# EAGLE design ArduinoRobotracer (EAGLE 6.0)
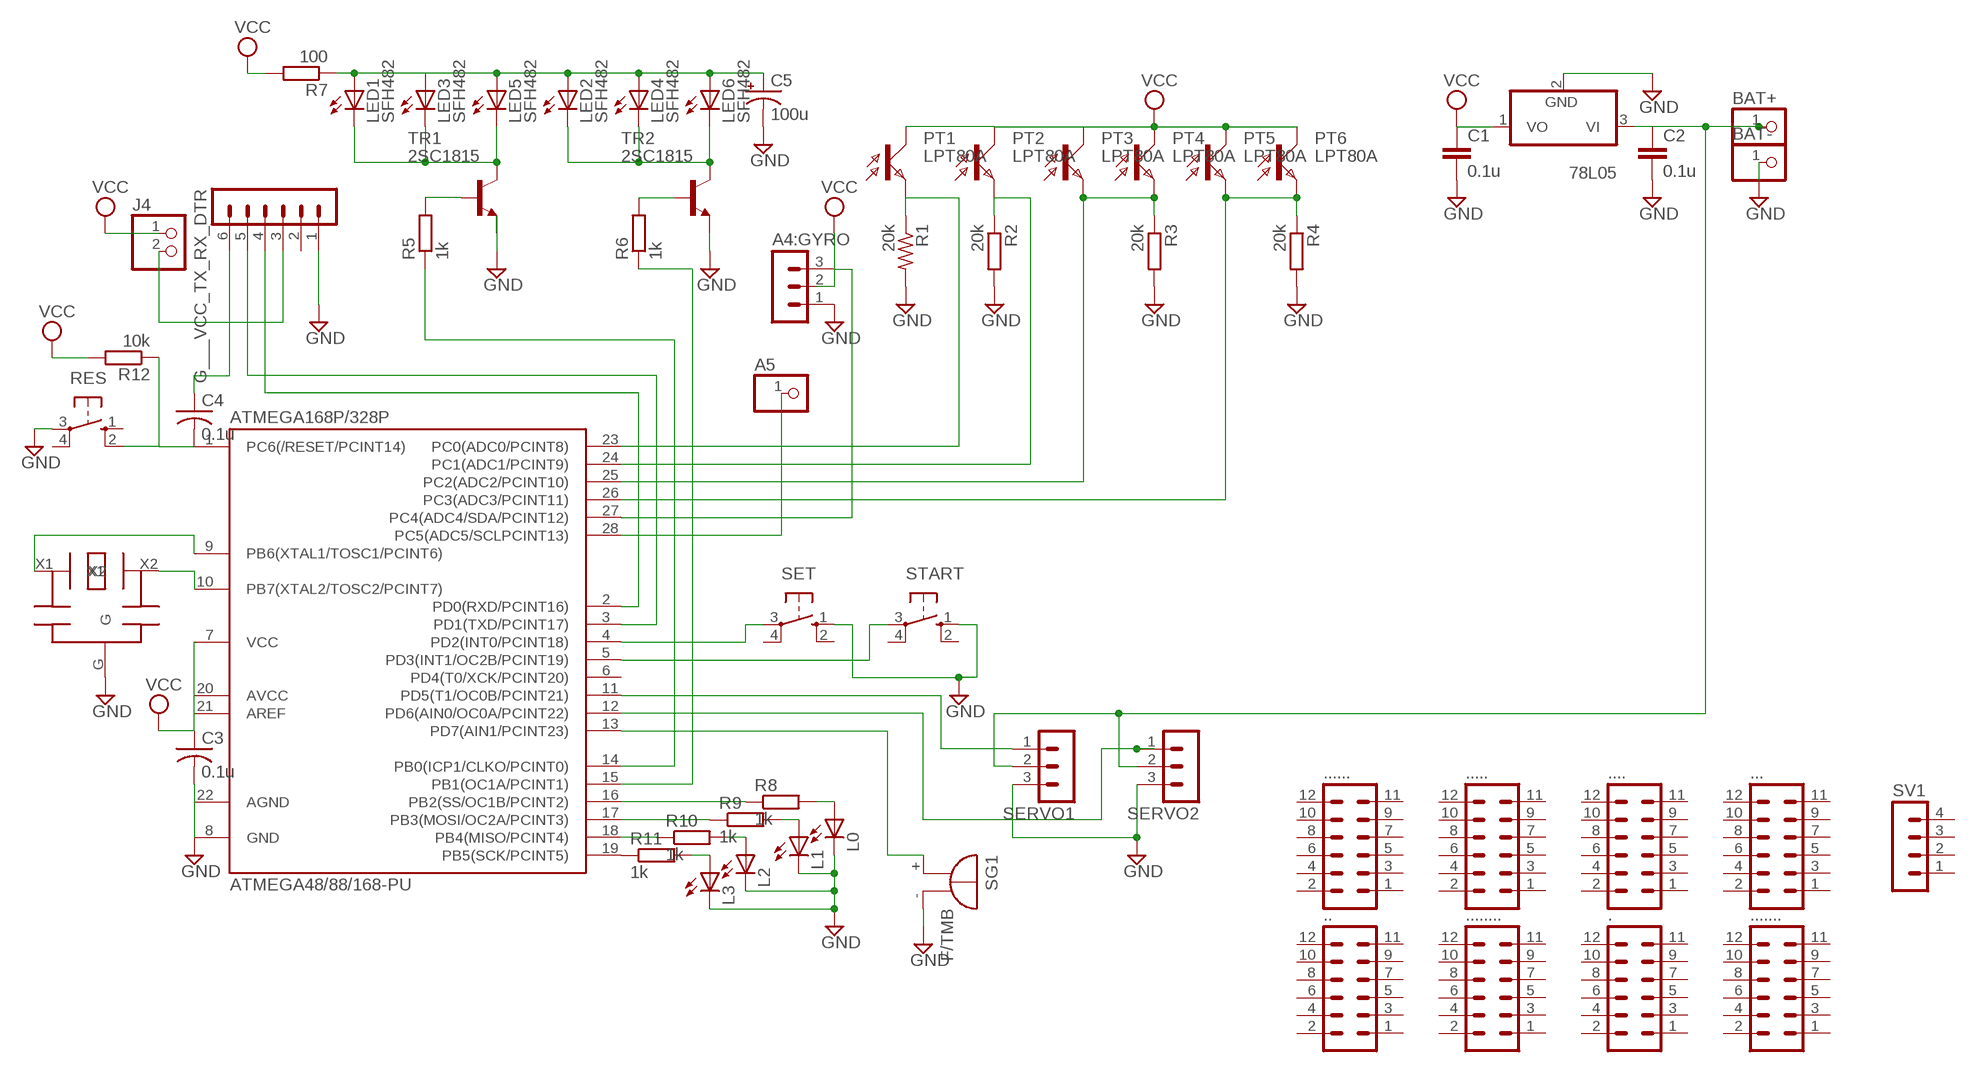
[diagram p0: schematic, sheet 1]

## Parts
78L05  78L05  [TO92-]
.  MA06-2  [MA06-2]
..  MA06-2  [MA06-2]
...  MA06-2  [MA06-2]
....  MA06-2  [MA06-2]
.....  MA06-2  [MA06-2]
......  MA06-2  [MA06-2]
.......  MA06-2  [MA06-2]
........  MA06-2  [MA06-2]
A4:GYRO  MA03-1  [MA03-1]
A5  PINHD-1X1  [1X01]
ATMEGA168P/328P  ATMEGA48/88/168-PU  [DIL28-3]
BAT+  PINHD-1X1  [1X01]
BAT-  PINHD-1X1  [1X01]
C1  0.1u  C2.5/2  [C2.5-2]
C2  0.1u  C2.5/2  [C2.5-2]
C3  0.1u  C-US025-025X050  [C025-025X050]
C4  0.1u  C-US025-025X050  [C025-025X050]
C5  100u  CPOL-USTT2D5  [TT2D5]
G___VCC_TX_RX_DTR  MA06-1  [MA06-1]
J4  PINHD-1X2  [1X02]
L0  LED3MM  [LED3MM]
L1  LED3MM  [LED3MM]
L2  LED3MM  [LED3MM]
L3  LED3MM  [LED3MM]
LED1  SFH482  [SFH482]
LED2  SFH482  [SFH482]
LED3  SFH482  [SFH482]
LED4  SFH482  [SFH482]
LED5  SFH482  [SFH482]
LED6  SFH482  [SFH482]
PT1  LPT80A  [LPT80A]
PT2  LPT80A  [LPT80A]
PT3  LPT80A  [LPT80A]
PT4  LPT80A  [LPT80A]
PT5  LPT80A  [LPT80A]
PT6  LPT80A  [LPT80A]
R1  20k  R-US_0204/2V  [0204V]
R2  20k  R-EU_0204/2V  [0204V]
R3  20k  R-EU_0204/2V  [0204V]
R4  20k  R-EU_0204/2V  [0204V]
R5  1k  R-EU_0204/2V  [0204V]
R6  1k  R-EU_0204/2V  [0204V]
R7  100  R-EU_0204/2V  [0204V]
R8  1k  R-EU_0204/2V  [0204V]
R9  1k  R-EU_0204/2V  [0204V]
R10  1k  R-EU_0204/2V  [0204V]
R11  1k  R-EU_0204/2V  [0204V]
R12  10k  R-EU_0204/2V  [0204V]
RES  10-XX  [B3F-10XX]
SERVO1  MA03-1  [MA03-1]
SERVO2  MA03-1  [MA03-1]
SET  10-XX  [B3F-10XX]
SG1  F/TMB  [F/TMB]
START  10-XX  [B3F-10XX]
SV1  MA04-1  [MA04-1]
TR1  2SC1815  [TO92-ECB]
TR2  2SC1815  [TO92-ECB]
U$1  CERALOCK  [CERALOCK]

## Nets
GND: 78L05.2(GND) A4:GYRO.1 ATMEGA168P/328P.8(GND) ATMEGA168P/328P.22(AGND) BAT-.1 C1.2 C2.2 C3.2 C5.- G___VCC_TX_RX_DTR.1 L0.K(C) L1.K(C) L2.K(C) L3.K(C) R1.2 R2.2 R3.2 R4.2 RES.3(P) SERVO1.3 SERVO2.3 SET.1(S) SG1.- START.1(S) TR1.E TR2.E U$1.G
N$1: ATMEGA168P/328P.25(PC2(ADC2/PCINT10)) PT3.E PT4.E R3.1
N$2: R5.2 TR1.B
N$3: ATMEGA168P/328P.18(PB4(MISO/PCINT4)) R10.1
N$4: A5.1 ATMEGA168P/328P.28(PC5(ADC5/SCLPCINT13))
N$5: ATMEGA168P/328P.4(PD2(INT0/PCINT18)) SET.3(P)
N$6: ATMEGA168P/328P.17(PB3(MOSI/OC2A/PCINT3)) R9.1
N$7: ATMEGA168P/328P.26(PC3(ADC3/PCINT11)) PT5.E PT6.E R4.1
N$8: ATMEGA168P/328P.24(PC1(ADC1/PCINT9)) PT2.E R2.1
N$9: ATMEGA168P/328P.16(PB2(SS/OC1B/PCINT2)) R8.1
N$10: ATMEGA168P/328P.1(PC6(/RESET/PCINT14)) C4.2 R12.1 RES.2(S1)
N$11: C5.+ LED1.A LED2.A LED3.A LED4.A LED5.A LED6.A R7.1
N$12: LED1.K(C) LED3.K(C) LED5.K(C) TR1.C
N$13: C4.1 G___VCC_TX_RX_DTR.6
N$14: LED2.K(C) LED4.K(C) LED6.K(C) TR2.C
N$15: ATMEGA168P/328P.19(PB5(SCK/PCINT5)) R11.1
N$16: L3.A R11.2
N$17: L2.A R10.2
N$18: ATMEGA168P/328P.2(PD0(RXD/PCINT16)) G___VCC_TX_RX_DTR.4
N$19: ATMEGA168P/328P.3(PD1(TXD/PCINT17)) G___VCC_TX_RX_DTR.5
N$20: L1.A R9.2
N$21: R6.2 TR2.B
N$22: ATMEGA168P/328P.5(PD3(INT1/OC2B/PCINT19)) START.3(P)
N$23: ATMEGA168P/328P.15(PB1(OC1A/PCINT1)) R6.1
N$24: L0.A R8.2
N$25: ATMEGA168P/328P.10(PB7(XTAL2/TOSC2/PCINT7)) U$1.X2
N$26: ATMEGA168P/328P.9(PB6(XTAL1/TOSC1/PCINT6)) U$1.X1
N$27: ATMEGA168P/328P.23(PC0(ADC0/PCINT8)) PT1.E R1.1
N$28: ATMEGA168P/328P.14(PB0(ICP1/CLKO/PCINT0)) R5.1
N$29: ATMEGA168P/328P.11(PD5(T1/OC0B/PCINT21)) SERVO1.1
N$30: G___VCC_TX_RX_DTR.3 J4.2
N$31: A4:GYRO.3 ATMEGA168P/328P.27(PC4(ADC4/SDA/PCINT12))
N$32: ATMEGA168P/328P.13(PD7(AIN1/PCINT23)) SG1.+
N$34: ATMEGA168P/328P.12(PD6(AIN0/OC0A/PCINT22)) SERVO2.1
N$35: 78L05.3(VI) BAT+.1 C2.1 SERVO1.2 SERVO2.2
VCC: 78L05.1(VO) A4:GYRO.2 ATMEGA168P/328P.7(VCC) ATMEGA168P/328P.20(AVCC) ATMEGA168P/328P.21(AREF) C1.1 C3.1 J4.1 PT1.C PT2.C PT3.C PT4.C PT5.C PT6.C R7.2 R12.2
Unconnected: ..1 ..2 ..3 ..4 ..5 ..6 ..7 ..8 ..9 ..10 ..11 ..12 ...1 ...2 ...3 ...4 ...5 ...6 ...7 ...8 ...9 ...10 ...11 ...12 ....1 ....2 ....3 ....4 ....5 ....6 ....7 ....8 ....9 ....10 ....11 ....12 .....1 .....2 .....3 .....4 .....5 .....6 .....7 .....8 .....9 .....10 .....11 .....12 ......1 ......2 ......3 ......4 ......5 ......6 ......7 ......8 ......9 ......10 ......11 ......12 .......1 .......2 .......3 .......4 .......5 .......6 .......7 .......8 .......9 .......10 .......11 .......12 ........1 ........2 ........3 ........4 ........5 ........6 ........7 ........8 ........9 ........10 ........11 ........12 .........1 .........2 .........3 .........4 .........5 .........6 .........7 .........8 .........9 .........10 .........11 .........12 ATMEGA168P/328P.6(PD4(T0/XCK/PCINT20)) G___VCC_TX_RX_DTR.2 RES.1(S) RES.4(P1) SET.2(S1) SET.4(P1) START.2(S1) START.4(P1) SV1.1 SV1.2 SV1.3 SV1.4

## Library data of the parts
78L05 = 1-linear:78*: Positive VOLTAGE REGULATOR
. .. ... .... ..... ...... ....... ........ = con-lstb:MA06-2: PIN HEADER; OC_FARNELL: unknown; OC_NEWARK: unknown
A4:GYRO SERVO1 SERVO2 = con-lstb:MA03-1: PIN HEADER
A5 BAT+ BAT- = pinhead:PINHD-1X1: PIN HEADER
ATMEGA168P/328P = atmega8:ATMEGA48/88/168-PU
C1 C2 = capacitor-wima:C: CAPACITOR
C3 C4 = resistor:C-US: CAPACITOR, American symbol
C5 = resistor:CPOL-US: POLARIZED CAPACITOR, American symbol
G___VCC_TX_RX_DTR = con-lstb:MA06-1: PIN HEADER
J4 = pinhead:PINHD-1X2: PIN HEADER
L0 L1-L3 = led:LED: LED
LED1-LED6 = led:SFH482: IR LED
PT1-PT6 = opto-trans-siemens:LPT80A: PHOTO TRANSISTOR
R1 = resistor:R-US_: RESISTOR, American symbol
R2-R6 = rcl:R-EU_: RESISTOR, European symbol
R7-R12 = resistor:R-EU_: RESISTOR, European symbol
RES SET START = switch-omron:10-XX: OMRON SWITCH
SG1 = buzzer:F/TMB: BUZZER; OC_FARNELL: unknown; OC_NEWARK: unknown
SV1 = con-lstb:MA04-1: PIN HEADER; OC_FARNELL: unknown; OC_NEWARK: unknown
TR1 TR2 = transistor:2SC1815: NPN EPITAXIAL TRANSISTOR Source: TOSHIBA .. 2SC1815 1.pdf
U$1 = ceralock:CERALOCK

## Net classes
1 +5V: width 0.61 mm, drill 0.406 mm
2 GND: width 0.914 mm, drill 0.406 mm

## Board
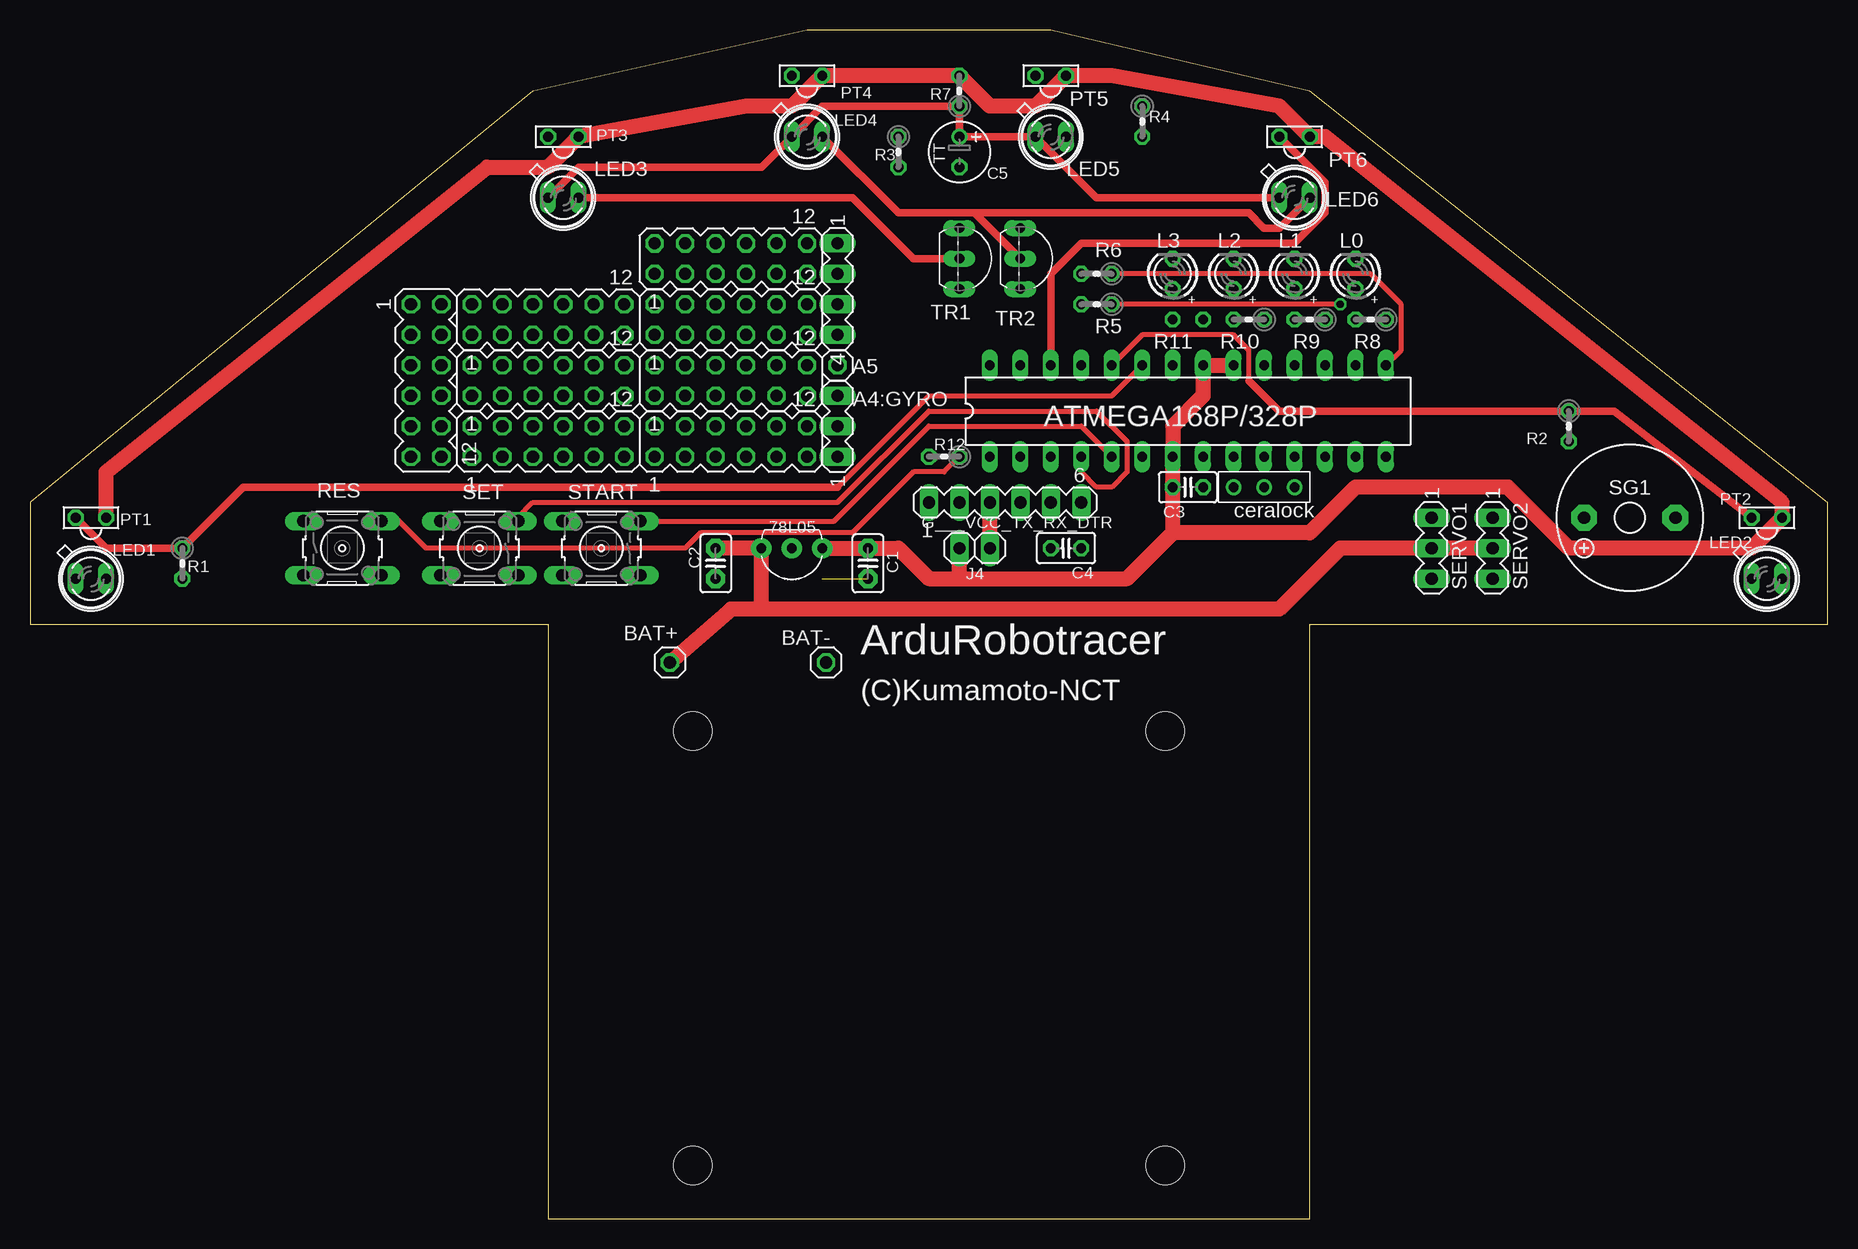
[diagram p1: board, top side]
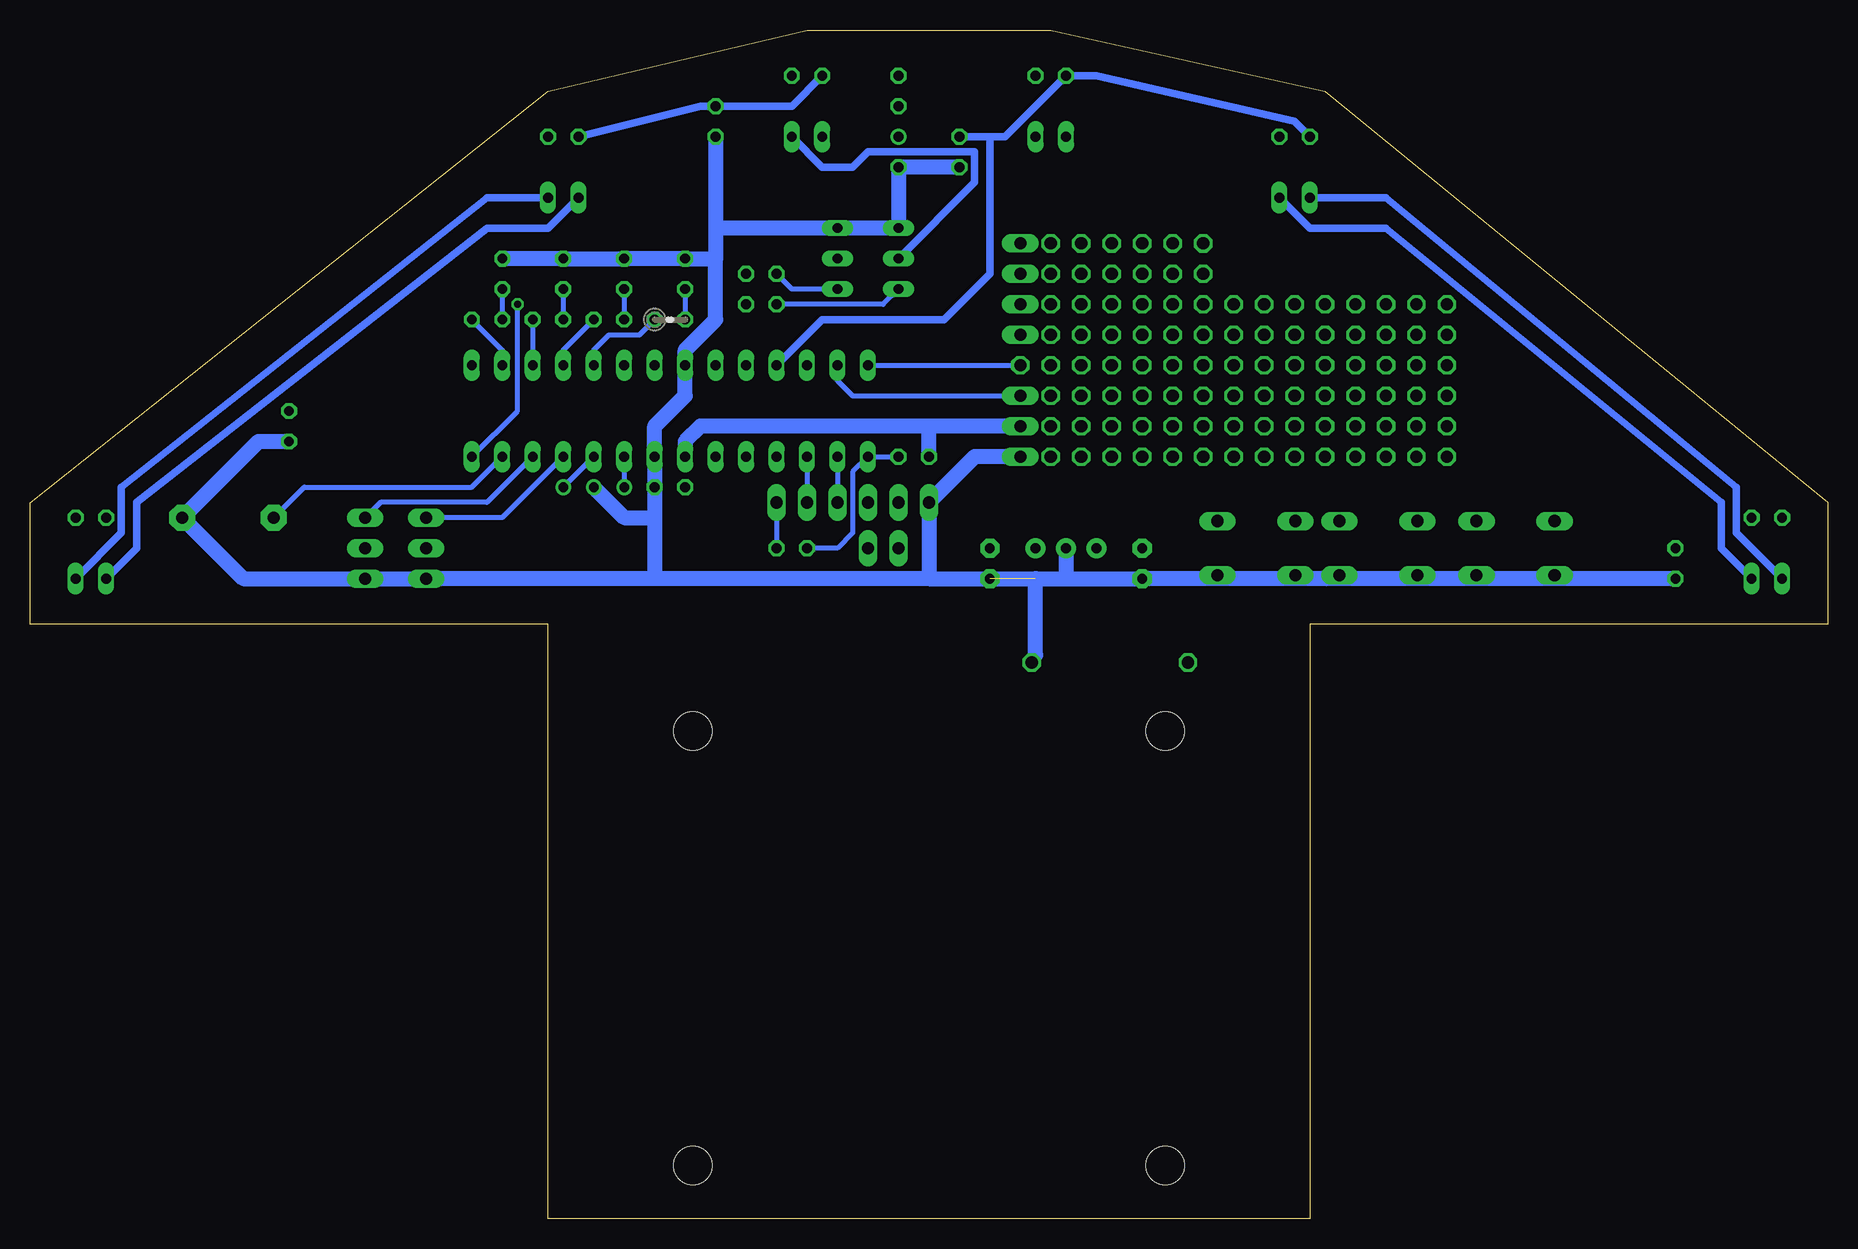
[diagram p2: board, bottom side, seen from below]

Size 149.86 x 99.06 mm. Coordinates in mm from the lower left corner, seen from the top.
Outline: 43.18,0 106.68,0 106.68,49.53 149.86,49.53 149.86,59.68 106.67,93.97 85.09,99.06 64.77,99.06 41.91,93.97 0,59.69 0,49.53 43.18,49.53 43.18,0
Copper layers (1*16): Top 0.035mm / dielectric 1.5mm / Bottom 0.035mm
Design rules: minimum track width 16mil, minimum drill 24mil, track to track 8mil, track to pad 8mil, pad to pad 8mil, via to via 8mil, smd to smd 8mil, copper to edge 40mil, drill to drill 8mil, minimum pad ring 10mil, minimum via ring 8mil, stop-mask expansion 4mil, vias tented up to drill 0mil, thermal gap 10mil
Holes 3.2 mm at 94.61,4.45 94.61,40.64 55.24,40.64 55.24,4.45

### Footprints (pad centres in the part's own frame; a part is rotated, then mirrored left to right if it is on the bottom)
TO92- = drill 0.813 pad 1.676: 1 -2.54,-1.27; 2 0,-1.27; 3 2.54,-1.27
MA06-2 = drill 1.016 octagon: 1 -6.35,-1.27; 2 -6.35,1.27; 3 -3.81,-1.27; 4 -3.81,1.27; 5 -1.27,-1.27; 6 -1.27,1.27; 7 1.27,-1.27; 8 1.27,1.27; 9 3.81,-1.27; 10 3.81,1.27; 11 6.35,-1.27; 12 6.35,1.27
MA03-1 = drill 1.016 long: 1 -2.54,0; 2 0,0; 3 2.54,0
1X01 = drill 1.016 octagon: 1 0,0
DIL28-3 = drill 0.813 long: 1 -16.51,-3.81; 2 -13.97,-3.81; 3 -11.43,-3.81; 4 -8.89,-3.81; 5 -6.35,-3.81; 6 -3.81,-3.81; 7 -1.27,-3.81; 8 1.27,-3.81; 9 3.81,-3.81; 10 6.35,-3.81; 11 8.89,-3.81; 12 11.43,-3.81; 13 13.97,-3.81; 14 16.51,-3.81; 15 16.51,3.81; 16 13.97,3.81; 17 11.43,3.81; 18 8.89,3.81; 19 6.35,3.81; 20 3.81,3.81; 21 1.27,3.81; 22 -1.27,3.81; 23 -3.81,3.81; 24 -6.35,3.81; 25 -8.89,3.81; 26 -11.43,3.81; 27 -13.97,3.81; 28 -16.51,3.81
C2.5-2 = drill 0.813 pad 1.6 octagon: 1 -1.27,0; 2 1.27,0
C025-025X050 = drill 0.813 octagon: 1 -1.27,0; 2 1.27,0
TT2D5 = drill 0.813: + -1.27,0 | drill 0.813 octagon: - 1.27,0
MA06-1 = drill 1.016 long: 1 -6.35,0; 2 -3.81,0; 3 -1.27,0; 4 1.27,0; 5 3.81,0; 6 6.35,0
1X02 = drill 1.016 long: 1 -1.27,0; 2 1.27,0
LED3MM = drill 0.813 octagon: A -1.27,0; K 1.27,0
SFH482 = drill 0.813 long: A -1.27,0; K 1.27,0
LPT80A = drill 0.813 octagon: C 0,-1.27; E 0,1.27
0204V = drill 0.813 octagon: 1 -1.27,0; 2 1.27,0
B3F-10XX = drill 1.016 long: 1 -3.251,2.261; 2 3.251,2.261; 3 -3.251,-2.261; 4 3.251,-2.261
F/TMB = drill 1.016 pad 2.159 octagon: + 3.81,0; - -3.81,0
MA04-1 = drill 1.016 long: 1 -3.81,0; 2 -1.27,0; 3 1.27,0; 4 3.81,0
TO92-ECB = drill 0.813 long: B 2.54,0; C 0,0; E -2.54,0
CERALOCK = drill 0.8: G 0,0; X1 -2.54,0; X2 2.54,0

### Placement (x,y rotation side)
78L05  63.5,54.61 180 top
.  33.02,69.85 270 top
..  43.18,74.93 0 top
...  43.18,69.85 0 top
....  43.18,64.77 0 top
.....  58.42,69.85 0 top
......  58.42,64.77 0 top
.......  58.42,80.01 0 top
........  58.42,74.93 0 top
A4:GYRO  67.31,66.04 90 top
A5  67.31,71.12 0 top
ATMEGA168P/328P  96.52,67.31 0 top
BAT+  53.34,46.35 0 top
BAT-  66.36,46.35 180 top
C1  69.85,54.61 270 top
C2  57.15,54.61 270 top
C3  96.52,60.96 0 top
C4  86.36,55.88 180 top
C5  77.47,88.9 270 top
G___VCC_TX_RX_DTR  81.28,59.69 0 top
J4  78.74,55.88 0 top
L0  110.49,78.74 90 top
L1  105.41,78.74 90 top
L2  100.33,78.74 90 top
L3  95.25,78.74 90 top
LED1  5.08,53.34 0 top
LED2  144.78,53.34 0 top
LED3  44.45,85.09 0 top
LED4  64.77,90.17 0 top
LED5  85.09,90.17 0 top
LED6  105.41,85.09 0 top
PT1  5.08,58.42 90 top
PT2  144.78,58.42 90 top
PT3  44.45,90.17 90 top
PT4  64.77,95.25 90 top
PT5  85.09,95.25 90 top
PT6  105.41,90.17 90 top
R1  12.7,54.61 270 top
R2  128.27,66.04 270 top
R3  72.39,88.9 270 top
R4  92.71,91.44 270 top
R5  88.9,76.2 180 top
R6  88.9,78.74 180 top
R7  77.47,93.98 90 top
R8  111.76,74.93 180 top
R9  106.68,74.93 180 top
R10  101.6,74.93 180 top
R11  96.52,74.93 0 bottom
R12  76.2,63.5 180 top
RES  26.04,55.88 0 top
SERVO1  116.84,55.88 270 top
SERVO2  121.92,55.88 270 top
SET  37.47,55.88 180 top
SG1  133.35,58.42 180 top
START  47.62,55.88 180 top
SV1  67.31,77.47 270 top
TR1  77.47,80.01 270 top
TR2  82.55,80.01 270 top
U$1  102.87,60.96 0 top

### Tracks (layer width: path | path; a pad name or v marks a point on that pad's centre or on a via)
GND  (1 unrouted)
  Bottom 0.406: RES.3 22.78,53.42 22.86,53.34 | 34.21,53.42 34.29,53.34 | 44.37,53.42 44.45,53.34 | 50.8,53.34 START.1
  Bottom 0.813: BAT-.1 66.04,46.99
  Bottom 1.27: R1.2 22.86,53.34 34.29,53.34 41.91,53.34 | 41.91,53.34 44.45,53.34 50.8,53.34 C2.2 63.5,53.34 | 74.93,53.34 97.79,53.34 | 97.79,53.34 SERVO1.3 SERVO2.3 132.08,53.34 SG1.- 130.81,64.77 R2.2 | 74.93,53.34 G___VCC_TX_RX_DTR.1 71.12,63.5 A4:GYRO.1 | U$1.G 100.33,58.42 97.79,58.42 | 97.79,58.42 97.79,53.34 | 97.79,58.42 C3.2 ATMEGA168P/328P.8 97.79,66.04 95.25,68.58 ATMEGA168P/328P.22 95.25,72.39 92.71,74.93 92.71,80.01 | L0.K L1.K L2.K L3.K 92.71,80.01 | 92.71,82.55 TR2.E TR1.E C5.- R3.2 | 92.71,82.55 92.71,80.01 | R4.2 92.71,82.55 | 74.93,53.34 66.04,53.34 | 66.04,53.34 63.5,53.34 | 41.91,53.34 SET.1 | 78L05.2 63.5,53.34 | 66.04,46.99 66.04,53.34
N$1
  Bottom 0.61: 69.85,90.17 68.58,90.17 PT4.E 60.96,95.25 44.45,91.44 PT3.E | ATMEGA168P/328P.25 83.82,74.93 73.66,74.93 69.85,78.74 69.85,90.17 | R3.1 69.85,90.17
N$2
  Bottom 0.406: TR1.B 78.74,76.2 R5.2
N$3
  Bottom 0.406: ATMEGA168P/328P.18 105.41,72.39 R10.1
N$4
  Bottom 0.406: ATMEGA168P/328P.28 A5.1
N$5
  Top 0.406: 40.72,58.5 41.91,59.69 67.31,59.69 74.93,67.31 88.9,67.31 91.44,64.77 91.44,62.23 90.17,60.96 88.9,60.96 87.63,62.23 ATMEGA168P/328P.4
  Top 0.61: SET.3 40.72,58.5
N$6
  Bottom 0.406: R9.1 ATMEGA168P/328P.17
N$7
  Top 0.61: ATMEGA168P/328P.26 85.09,78.74 87.63,81.28 105.41,81.28 107.95,83.82 107.95,86.36 PT6.E
  Bottom 0.61: PT6.E 93.98,92.71 R4.1 86.36,92.71 PT5.E
N$8
  Top 0.406: ATMEGA168P/328P.24 92.71,73.66 100.33,73.66 101.6,72.39 101.6,69.85
  Top 0.61: 101.6,69.85 104.14,67.31 R2.1 132.08,67.31 PT2.E
N$9
  Bottom 0.406: R8.1 110.49,72.39 ATMEGA168P/328P.16
N$10
  Top 0.406: R12.1 76.2,62.23 73.66,62.23 68.58,57.15 55.88,57.15 54.61,55.88 33.02,55.88 30.48,58.42 RES.2
  Bottom 0.406: C4.2 82.55,55.88 81.28,57.15 81.28,62.23 ATMEGA168P/328P.1 R12.1
N$11
  Top 0.61: LED6.A 88.9,85.09 LED5.A C5.+ R7.1 66.04,92.71 LED4.A 60.96,87.63 45.72,87.63 LED3.A
  Bottom 0.61: LED1.A 7.62,57.15 7.62,60.96 36.83,85.09 LED3.A | LED2.A 140.97,55.88 140.97,59.69 111.76,82.55 106.68,82.55 LED6.A
N$12
  Top 0.61: TR1.C 73.66,80.01 68.58,85.09 LED3.K
  Bottom 0.61: LED1.K 8.89,55.88 8.89,59.69 36.83,82.55 43.18,82.55 LED3.K | LED5.K 83.82,87.63 81.28,87.63 80.01,88.9 71.12,88.9 71.12,86.36 TR1.C
N$13
  Bottom 0.406: G___VCC_TX_RX_DTR.6 C4.1
N$14
  Top 0.61: TR2.C 78.74,83.82 | LED6.K 104.14,82.55 102.87,82.55 101.6,83.82 78.74,83.82 | LED4.K 72.39,83.82 78.74,83.82
  Bottom 0.61: LED2.K 142.24,57.15 142.24,60.96 111.76,85.09 LED6.K
N$15
  Bottom 0.406: ATMEGA168P/328P.19 102.87,72.39 101.6,73.66 99.06,73.66 R11.1
N$16
  Bottom 0.406: L3.A R11.2
N$17
  Bottom 0.406: L2.A R10.2
N$18
  Bottom 0.406: ATMEGA168P/328P.2 G___VCC_TX_RX_DTR.4
N$19
  Bottom 0.406: ATMEGA168P/328P.3 G___VCC_TX_RX_DTR.5
N$20
  Bottom 0.406: L1.A R9.2
N$21
  Bottom 0.406: TR2.B 86.36,77.47 R6.2
N$22
  Top 0.406: START.3 67.03,58.14 74.93,66.04 87.63,66.04 ATMEGA168P/328P.5
N$23
  Top 0.406: R6.1 111.76,78.74 114.3,76.2 114.3,72.39 ATMEGA168P/328P.15
N$24
  Bottom 0.406: L0.A R8.2
N$25
  Bottom 0.406: ATMEGA168P/328P.10 U$1.X2
N$26
  Bottom 0.406: ATMEGA168P/328P.9 U$1.X1
N$27
  Top 0.406: 67.31,60.96 74.93,68.58 90.17,68.58 ATMEGA168P/328P.23
  Top 0.61: PT1.E 6.35,55.88 R1.1 17.78,60.96 67.31,60.96
N$28  (via drill 0.61)
  Top 0.406: v109.22,76.2 R5.1
  Bottom 0.406: v109.22,76.2 109.22,67.31 ATMEGA168P/328P.14
N$29
  Bottom 0.406: ATMEGA168P/328P.11 110.49,58.42 SERVO1.1
N$30
  Top 1.27: J4.2 G___VCC_TX_RX_DTR.3
N$31
  Bottom 0.406: ATMEGA168P/328P.27 82.55,69.85 81.28,68.58 A4:GYRO.3
N$32
  Bottom 0.406: ATMEGA168P/328P.13 113.03,60.96 127,60.96 SG1.+
N$34
  Bottom 0.406: ATMEGA168P/328P.12 111.76,59.69 120.65,59.69 SERVO2.1
N$35
  Top 1.27: SERVO2.2 SERVO1.2 109.22,55.88 104.14,50.8 60.96,50.8 | 60.96,50.8 58.42,50.8 BAT+.1 | 60.96,50.8 78L05.3 C2.1
VCC
  Top 1.27: 77.47,53.34 91.44,53.34 95.25,57.15 | 95.25,57.15 C3.1 ATMEGA168P/328P.7 95.25,66.04 97.79,68.58 ATMEGA168P/328P.21 ATMEGA168P/328P.20 | 77.47,53.34 74.93,53.34 72.39,55.88 C1.1 78L05.1 | 77.47,53.34 J4.1 | 95.25,57.15 106.68,57.15 110.49,60.96 123.19,60.96 128.27,55.88 143.51,55.88 PT2.C 146.05,59.69 107.95,90.17 PT6.C 104.14,92.71 90.17,95.25 PT5.C 83.82,92.71 80.01,92.71 R7.2 PT4.C 63.5,92.71 59.69,92.71 PT3.C 43.18,87.63 38.1,87.63 6.35,62.23 PT1.C
  Bottom 1.27: A4:GYRO.2 74.93,66.04 | 74.93,66.04 93.98,66.04 95.25,64.77 ATMEGA168P/328P.7 | R12.2 74.93,66.04

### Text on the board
tPlace: + | + | + | + | ArduRobotracer | (C)Kumamoto-NCT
